FUNCTION_BLOCK FB_DO_IED_LD1_LEDGGIO5_NamPlt EXTENDS FB_AcsiCommonDataClass
VAR_INPUT
	vendor: FB_AcsiDATypeVisString255 := (fc:=ACSI_FC_DC, sValue:='Beckhoff Automation', bLinkResult:=THIS^.AddDataToContainer(ipData:=vendor));
	swRev: FB_AcsiDATypeVisString255 := (fc:=ACSI_FC_DC, sValue:='1.0', bLinkResult:=THIS^.AddDataToContainer(ipData:=swRev));
	d: FB_AcsiDATypeVisString255 := (fc:=ACSI_FC_DC, sValue:='Demo LED output 5', bLinkResult:=THIS^.AddDataToContainer(ipData:=d));
END_VAR
VAR
END_VAR

END_FUNCTION_BLOCK
